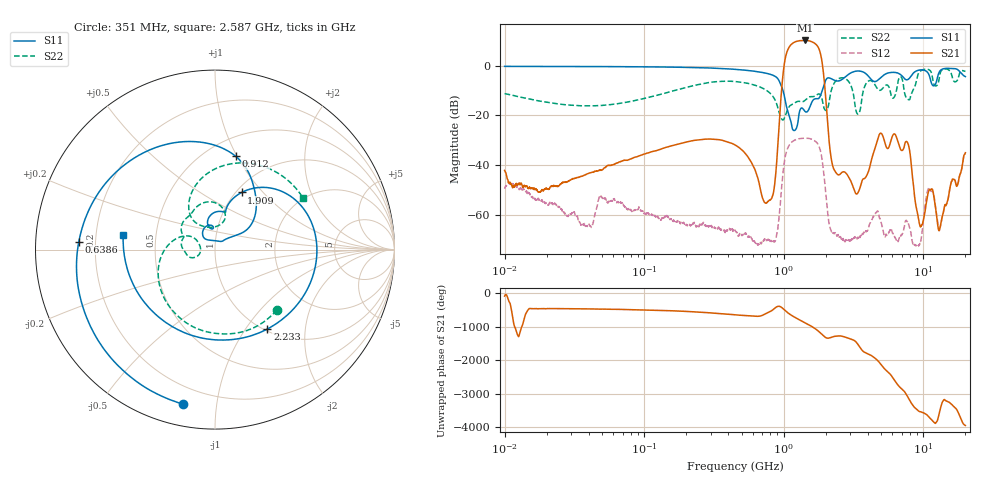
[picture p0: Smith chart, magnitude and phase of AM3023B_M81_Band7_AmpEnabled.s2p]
!Agilent Technologies,E8364B,MY43040894,A.07.50.67
!Agilent E8364B: A.07.50.67
!Date: Tuesday, October 27, 2020 10:44:28
!Correction: S11(Full 2 Port(1,2))
!S21(Full 2 Port(1,2))
!S12(Full 2 Port(1,2))
!S22(Full 2 Port(1,2))
!S2P File: Measurements: S11, S21, S12, S22:Log Frequency Sweep
# Hz S  dB  R 50
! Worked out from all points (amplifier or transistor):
!   3201 points, 10 MHz to 20 GHz, reference 50 ohm
!   highest |S21| = 10.1 dB at 1.419 GHz (marker M1)
!   |S21| within 3 dB of that: 1.085 GHz to 1.774 GHz (689.5 MHz wide, 48.2 % of centre)
!   unconditionally stable (mu >= 1): start of sweep to end of sweep
!   at 35.47 MHz: K = 11001.63, MAG = -33.6 dB, |S12| = -64.2 dB
!   at 447.2 MHz: K = 8990.71, MAG = -25.4 dB, |S12| = -66.2 dB
!   at 20 GHz: K = 441.82, MAG = -29.3 dB, |S12| = -35.4 dB
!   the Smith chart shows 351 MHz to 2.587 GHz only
!   S11 on the Smith chart (normalised r, x): 351 MHz: 0.11, -0.81; 638.6 MHz: 0.14, +0.03; 912 MHz: 0.68, +0.99; 1.909 GHz: 1.06, +0.77; 2.233 GHz: 1.03, -1.27; 2.587 GHz: 0.32, +0.07
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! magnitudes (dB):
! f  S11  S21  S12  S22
! 10 MHz  -0.3  -42.2  -49.6  -11.3
! 35.55 MHz  -0.4  -44.6  -64.2  -16.2
! 49.34 MHz  -0.4  -42.1  -52.7  -16.0
! 126.1 MHz  -0.5  -34.0  -61.4  -11.8
! 351 MHz  -1.1  -29.9  -65.7  -6.3
! 447.2 MHz  -1.5  -31.9  -66.2  -6.4
! 638.6 MHz  -2.4  -43.7  -72.3  -8.1
! 809.9 MHz  -3.6  -53.8  -70.6  -11.5
! 912 MHz  -5.5  -30.0  -64.4  -17.6
! 1.047 GHz  -16.6  5.0  -34.5  -18.8
! 1.419 GHz  -18.4  10.1  -29.2  -14.0
! 1.59 GHz  -14.7  9.6  -29.7  -12.5
! 1.909 GHz  -9.1  -1.3  -40.6  -15.4
! 2.233 GHz  -5.5  -40.0  -67.4  -8.5
! 2.587 GHz  -5.7  -43.2  -70.0  -4.9
! 3.392 GHz  -2.2  -51.3  -69.1  -19.6
! 5.639 GHz  -2.9  -33.1  -67.2  -8.4
! 7.716 GHz  -5.6  -31.1  -63.1  -13.5
! 9.623 GHz  -1.7  -64.5  -70.1  -2.0
! 10.84 GHz  -3.1  -51.1  -49.7  -1.5
! 13.14 GHz  -2.2  -65.5  -65.2  -3.4
! 20 GHz  -4.4  -35.1  -35.4  -2.3
